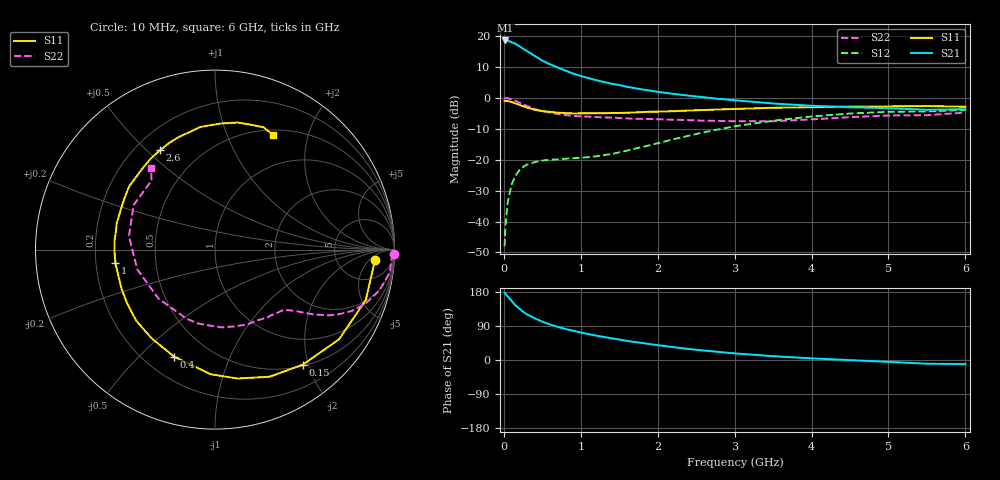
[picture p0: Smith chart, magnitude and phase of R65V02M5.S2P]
! SIEMENS Small Signal Semiconductors
! BFR193
! Si NPN RF Bipolar Junction Transistor in SOT23
! VCE = 5 V  IC = 2.5 mA
! Common Emitter S-Parameters:  May  1996
# GHz  S  MA  R  50
!  f  S11  S21  S12  S22
! GHz  MAG  ANG  MAG  ANG  MAG  ANG  MAG  ANG
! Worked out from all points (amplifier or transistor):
!   36 points, 10 MHz to 6 GHz, reference 50 ohm
!   highest |S21| = 18.5 dB at 20 MHz (marker M1)
!   |S21| within 3 dB of that: start of sweep to 271.4 MHz
!   unconditionally stable (mu >= 1): 1.108 GHz to 2.038 GHz
!   at 250 MHz: K = 0.27, MSG = 19.1 dB, |S12| = -22.4 dB
!   at 1.4 GHz: K = 1.09, MAG = 9.5 dB, |S12| = -18.2 dB
!   at 6 GHz: K = 0.99, MSG = 0.1 dB, |S12| = -3.9 dB
!   S11 on the Smith chart (normalised r, x): 10 MHz: 13, -8; 150 MHz: 0.52, -1.91; 400 MHz: 0.32, -0.64; 1 GHz: 0.28, -0.06; 2.6 GHz: 0.30, +0.55; 6 GHz: 0.57, +1.48
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0.01  0.8926 -3.7  8.271 177.8  0.004 87.0  0.9971 -1.4
0.02  0.8859 -7.5  8.417 174.9  0.0082 89.5  0.985 -2.9
0.05  0.8859 -18.5  8.343 167.7  0.0204 80.6  0.9825 -7.4
0.1  0.8528 -35.9  7.887 156.3  0.0394 71.8  0.9443 -13.9
0.15  0.8063 -52.7  7.461 144.6  0.0547 62.8  0.8907 -19.8
0.2  0.7708 -66.8  6.805 135.8  0.0669 56.5  0.8361 -24.1
0.25  0.7291 -80.1  6.18 127.6  0.076 51.1  0.7843 -27.2
0.3  0.6948 -92.0  5.675 120.5  0.0831 47.4  0.7366 -29.8
0.4  0.6386 -110.8  4.752 110.1  0.0908 41.6  0.6587 -33.3
0.5  0.6077 -125.4  3.97 101.2  0.0965 38.5  0.608 -35.3
0.6  0.5915 -137.9  3.473 93.8  0.0997 36.8  0.5747 -36.8
0.7  0.5737 -148.6  3.081 87.4  0.1011 36.9  0.5469 -38.4
0.8  0.5649 -157.3  2.739 82.0  0.1034 37.6  0.5253 -39.9
1  0.5598 -172.5  2.246 72.6  0.107 41.1  0.5015 -43.2
1.1  0.5602 -179.0  2.075 68.4  0.11 43.4  0.4946 -45.4
1.6  0.5721 155.4  1.504 50.5  0.1399 56.4  0.4633 -57.5
2.2  0.6054 132.4  1.155 34.0  0.2124 62.2  0.4404 -76.7
2.6  0.6327 119.1  1.018 25.0  0.2762 60.0  0.4248 -93.0
3.5  0.6884 96.7  0.807 10.1  0.4253 45.9  0.4167 -139.1
4.5  0.7191 79.9  0.701 -0.3  0.5561 26.1  0.4853 171.1
5.5  0.7332 68.3  0.64 -9.8  0.601 7.1  0.5227 132.6
6  0.7149 62.9  0.653 -10.9  0.6362 1.8  0.5755 128.2
